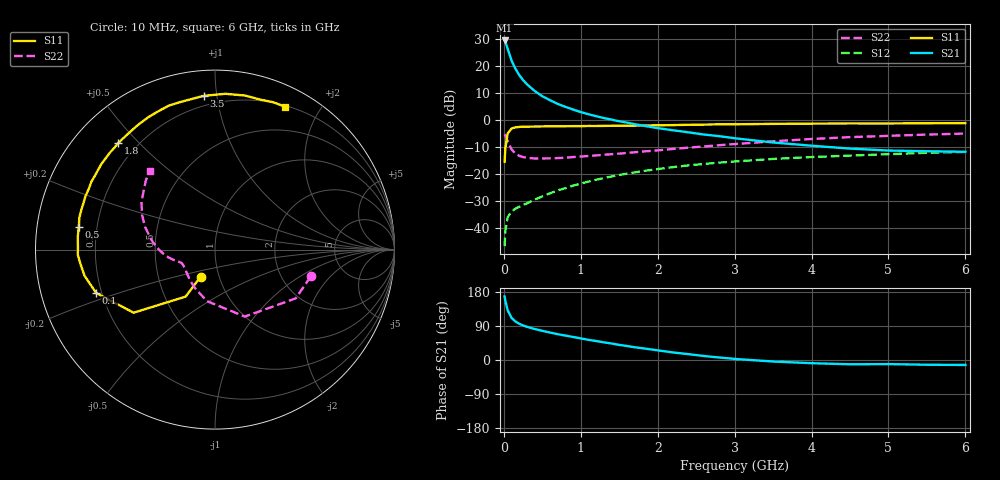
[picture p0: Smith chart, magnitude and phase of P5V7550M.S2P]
! SIEMENS Small Signal Semiconductors
! BFP183
! Si NPN RF Bipolar Junction Transistor in SOT143
! VCE = 0.75 V  IC = 50 mA
! Common Emitter S-Parameters:  March  1996
# GHz  S  MA  R  50
!  f  S11  S21  S12  S22
! GHz  MAG  ANG  MAG  ANG  MAG  ANG  MAG  ANG
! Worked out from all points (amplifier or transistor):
!   36 points, 10 MHz to 6 GHz, reference 50 ohm
!   highest |S21| = 29.5 dB at 10 MHz (marker M1)
!   |S21| within 3 dB of that: start of sweep to 48.51 MHz
!   unconditionally stable (mu >= 1): start of sweep to 33.05 MHz; 135.9 MHz to end of sweep
!   at 250 MHz: K = 1.39, MAG = 19.4 dB, |S12| = -31.3 dB
!   at 1.4 GHz: K = 2.01, MAG = 4.8 dB, |S12| = -20.8 dB
!   at 6 GHz: K = 1.56, MAG = -4.4 dB, |S12| = -11.7 dB
!   S11 on the Smith chart (normalised r, x): 10 MHz: 0.82, -0.25; 100 MHz: 0.18, -0.17; 500 MHz: 0.13, +0.08; 1.8 GHz: 0.13, +0.44; 3.5 GHz: 0.14, +0.92; 6 GHz: 0.21, +1.59
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0.01  0.1704 -117.9  30 167.6  0.0047 62.6  0.5538 -15.7
0.02  0.3087 -122.0  28.31 156.1  0.009 59.9  0.5257 -31.1
0.05  0.5736 -142.2  20.92 130.9  0.0162 48.6  0.4086 -66.0
0.1  0.7046 -159.9  12.79 111.2  0.0206 37.5  0.2905 -99.0
0.15  0.7412 -168.6  8.988 101.6  0.0232 38.0  0.242 -117.4
0.2  0.7543 -174.0  6.86 95.6  0.0252 39.6  0.2204 -129.1
0.25  0.7648 -177.8  5.544 91.2  0.0271 42.4  0.2088 -136.6
0.3  0.7636 179.2  4.639 87.6  0.0291 46.0  0.2021 -142.1
0.4  0.7677 174.7  3.494 81.8  0.0341 49.9  0.1973 -148.9
0.5  0.7697 170.4  2.794 77.0  0.0391 52.5  0.197 -153.1
0.6  0.7763 166.8  2.355 72.4  0.0447 54.8  0.1982 -155.8
0.7  0.7769 163.6  2.014 68.2  0.0506 56.5  0.2004 -157.8
0.9  0.7808 157.6  1.582 60.8  0.0619 57.5  0.2092 -160.4
1.1  0.7859 151.2  1.295 53.2  0.0737 57.3  0.2189 -162.8
1.5  0.7935 140.1  0.959 39.9  0.0974 54.6  0.242 -167.0
1.8  0.8021 132.1  0.802 31.0  0.1146 51.7  0.2647 -170.7
2.2  0.816 122.0  0.654 19.9  0.1363 46.8  0.2955 -176.8
2.8  0.8422 107.8  0.509 6.6  0.1648 39.0  0.3465 173.6
3.5  0.859 94.2  0.389 -4.0  0.1929 30.4  0.4089 162.2
4.5  0.8746 79.0  0.3 -11.3  0.2226 18.7  0.4887 146.9
5.5  0.8828 68.5  0.268 -12.5  0.2508 8.8  0.5451 135.0
6  0.8869 63.8  0.262 -13.1  0.2602 3.5  0.5688 129.6
